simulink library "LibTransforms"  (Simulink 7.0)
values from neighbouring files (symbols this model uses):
  a0 = 0.0    (= 0)    [quake.m]    (also in rampth.m = omega^3; rspect.m = 1; displA2T.m = positT2A(zeros(ntbl, 1), dof, rh, rb, rl, canon, atype); displEnvelope.m = varargin{1}{7})
  atype = []    [displA2T.m]    (also in displEnvelope.m = varargin{1}{6}; displJacobian.m = ones(nact, 1); displT2A.m; forceA2T.m)
  canon = [linDisplCanon linVelocCanon linAccelCanon linForceCanon  		 rotDisplCanon rotVelocCanon rotAccelCanon rotForceCanon]'    [initialize.m]    (also in accelEnvelope.m = varargin{1}{4}; displEnvelope.m = varargin{1}{5}; displPivotEnvelope.m = varargin{1}{6}; forceEnvelope.m = varargin{1}{6})
  dmax = ( (stroke2 + endLength2) * lengthCanon)'    [initialize.m]
  dof = [1 2]    [initialize.m]    (also in accelEnvelope.m = varargin{1}{1}; displEnvelope.m = varargin{1}{1}; displPivotEnvelope.m = varargin{1}{1}; forceEnvelope.m = varargin{1}{2})
  ea = dcm * ea    [initialize.m]    (also in accelEnvelope.m = varargin{1}{3})
  fmax = ( area1 * areaCanon * (supplyPress-returnPress) * pressCanon)'    [initialize.m]    (also in Tutorial.m = 50; forceEnvelope.m = varargin{1}{10}; forceJacobian.m = []; forceT2A.m = [])
  gee = geeCanon / linAccelCanon * 0    (= 0)    [initialize.m]    (also in accelA2T.m; accelEnvelope.m = varargin{1}{6}; accelT2A.m)
  linAccelCanon = 9810.0    (= 9810)    [initialize.m]    (also in accelJacobian.m = canon(3); accelP2Q.m = canon(3))
  linDisplCanon = 1    [initialize.m]    (also in displJacobian.m = canon(1); velocJacobian.m = canon(1))
  linVelocCanon = 1000.0    (= 1000)    [initialize.m]    (also in forceInvJacobian.m = canon(2); velocJacobian.m = canon(2); velocP2Q.m = canon(2))
  ra = dcm * ra    [initialize.m]    (also in accelEnvelope.m = varargin{1}{2})
  rb = dcm * rb    [initialize.m]    (also in displEnvelope.m = varargin{1}{3}; displPivotEnvelope.m = varargin{1}{3}; forceEnvelope.m = varargin{1}{4}; velocEnvelope.m = varargin{1}{4})
  rh = dcm * rh    [initialize.m]    (also in displEnvelope.m = varargin{1}{2}; displPivotEnvelope.m = varargin{1}{2}; forceEnvelope.m = varargin{1}{3}; velocEnvelope.m = varargin{1}{3})
  rl = dcm * rl    [initialize.m]    (also in displEnvelope.m = varargin{1}{4}; displPivotEnvelope.m = varargin{1}{4}; forceEnvelope.m = varargin{1}{5}; velocEnvelope.m = varargin{1}{5})
  rotAccelCanon = pi/180    (= 0.0174532925199)    [initialize.m]    (also in accelJacobian.m = canon(7); accelP2Q.m = canon(7); bodyAccel.m = canon(3); eulerAccel.m = canon(3))
  rotDisplCanon = pi/180    (= 0.0174532925199)    [initialize.m]    (also in accelA2T.m = canon(5); accelP2Q.m = canon(5); accelT2A.m = canon(5); bodyAccel.m = canon(1))
  rotForceCanon = 1000    [initialize.m]    (also in forceInvJacobian.m = canon(8); forceP2Q.m = canon(8))
  rotVelocCanon = pi/180    (= 0.0174532925199)    [initialize.m]    (also in accelJacobian.m = canon(6); accelP2Q.m = canon(6); bodyAccel.m = canon(2); eulerAccel.m = canon(2))
  rows = size(header, 1)    [player.m]    (also in quake.m; savebin.m; viewer.m; accelA2T.m = size(vrot, 1))
  rpq = rpq(:)    [accelP2Q.m]    (also in displP2Q.m; forceP2Q.m; velocP2Q.m)
undefined symbols (not defined in the file or in its folder): aijac, ajac, cols, Column, D, magnitude, matrix, vector
libraries: LibTransforms x99, aerospace x9, simulink x6
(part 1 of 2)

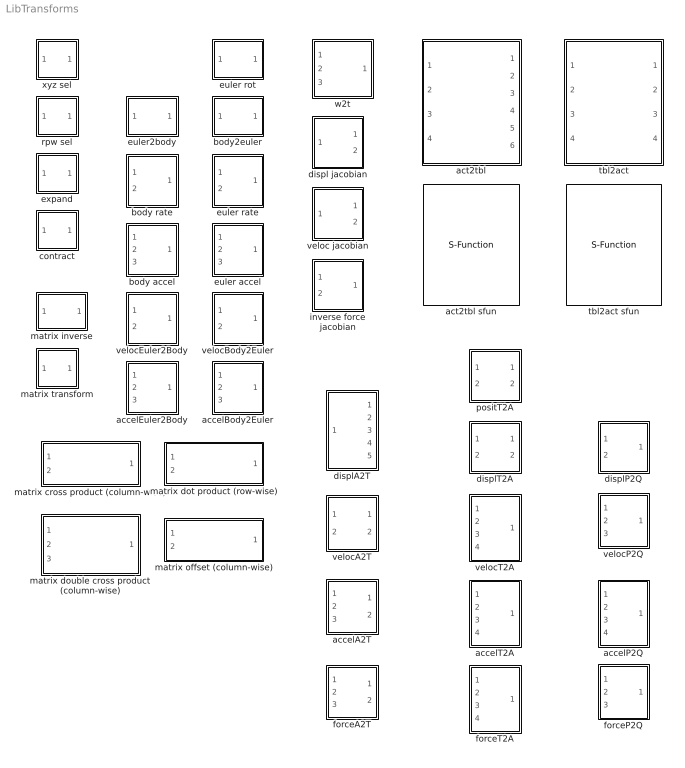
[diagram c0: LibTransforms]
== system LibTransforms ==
  accelA2T : Subsystem  mask(Accelerometer values to table acceleration tranform){dof=dof, ra=ra, ea=ea, ijac=aijac, gee=gee}
      mask prompts: dof "Degree-of-freedom indices"; ra "Accelerometer location vectors"; ea "Accelerometer orientation vectors"; ijac "Inverse acceleration jacobian"; gee "Gravity constant"
  accelBody2Euler : Subsystem  mask(Body acceleration to euler acceleration transform){dof=dof}
      mask prompts: dof "Degree-of-freedom indices"
  accelEuler2Body : Subsystem  mask(Euler acceleration to body acceleration transform){dof=dof}
      mask prompts: dof "Degree-of-freedom indices"
  accelP2Q : Subsystem  mask(Origin offset acceleration transform){dof=dof, ofst=rpq}
      mask prompts: dof "Degree-of-freedom indices"; ofst "Origin offset vector"
  accelT2A : Subsystem  mask(Table acceleration to accelerometer values tranform){dof=dof, ra=ra, ea=ea, jac=ajac, gee=gee}
      mask prompts: dof "Degree-of-freedom indices"; ra "Accelerometer location vectors"; ea "Accelerometer orientation vectors"; jac "Acceleration jacobian"; gee "Gravity constant"
  act2tbl : Subsystem  mask(Actuator to table transform){dof=dof, rh=rh, rb=rb, a0=a0, ra=ra, ea=ea, aijac=aijac, fmax=fmax, gee=gee}
      mask prompts: dof "Degree-of-freedom indices"; rh "Table pivot location vectors"; rb "Base pivot location vectors"; a0 "Actuator home position"; ra "Acceleration location vectors"; ea "Acceleration orientation vectors"; aijac "Inverse acceleration jacobian"; fmax "Actuator max forces"; gee "Gravity constant"
  act2tbl sfun : S-Function  FunctionName=Act2Tbl  Parameters=atype, nVel, nFrc, dof, rh, rb, rl, ra, ea, offset, dmax, fmax, canon, gee, action, rate, count  mask(Actuator-to-table transform){atype=atype, nVel=length(atype), nFrc=length(atype), dof=dof, rh=rh, rb=rb, rl=rl, ra=ra, ea=ea, offset=[0 0 0 0 0 0], dmax=dmax, fmax=fmax, canon=canon, gee=gee, action=1, rate=1, count=1}
      mask prompts: atype "Actuator types (1: inline; 2: pedestal-link; 3: sliding head; 4: sliding base)"; nVel "Number of velocity sensors (0 or nAct)"; nFrc "Number of force sensors (0 or nAct)"; dof "Degree-of-freedom indices (1: X; 2: Y; 3: Z; 4: Roll; 5: Pitch; 6: Yaw)"; rh "Head pivot location vectors"; rb "Base pivot location vectors"; rl "Link pivot location vectors"; ra "Accelerometer location vectors"; ea "Accelerometer orientation vectors"; offset "Coordinate system offset/rotation"; dmax "Actuator max displacements"; fmax "Actuator max forces"; canon "Canonical units"; gee "Gravity constant"; action "Jacobian update mode (0:static; 1: dyamic)"; rate "Rate type (0:body; 1:euler)"; count "Iteration count"
      mask init:
      | if nVel
      | 	velocInpName = 'velocA';
      | else
      | 	velocInpName = 'rot veloc';
      | end
  body accel : Subsystem
  body rate : Subsystem
  body2euler : Subsystem
  contract : Subsystem  mask(Linear degrees-of-freedom selector){elements=[1]}
      mask init:
      | if isempty(elements)
      | 	elements = 1;
      | end
  displ jacobian : Subsystem  mask(Displacement jacobian){dof=dof, rh=rh, rb=rb}
      mask prompts: dof "Degree-of-freedom indices"; rh "Table pivot location vectors"; rb "Base pivot location vectors"
  displA2T : Subsystem  mask(Actuator displacement to table displacement transform){dof=dof, rh=rh, rb=rb, a0=a0}
      mask prompts: dof "Degree-of-freedom indices"; rh "Table pivot location vectors"; rb "Base pivot location vectors"; a0 "Actuator home position"
  displP2Q : Subsystem  mask(Origin offset displacement transform){dof=dof, ofst=rpq}
      mask prompts: dof "Degree-of-freedom indices"; ofst "Origin offset vector"
  displT2A : Subsystem  mask(Table displacement to actuator displacement  transform){dof=dof, rh=rh, rb=rb, a0=a0}
      mask prompts: dof "Degree-of-freedom indices"; rh "Table pivot location vectors"; rb "Base pivot location vectors"; a0 "Actuator home position"
  euler accel : Subsystem
  euler rate : Subsystem
  euler rot : Subsystem
  euler2body : Subsystem
  expand : Subsystem  mask(Vector expander){size=6, elements=dof}
      mask prompts: size "Output vector size"; elements "Output vector elements (-1 for all elements)"
      mask init:
      | noElements = isempty(elements);
      | if noElements
      | 	elements = 1;
      | end
  forceA2T : Subsystem  mask(Actuator force to table force transform){dof=dof, rh=rh}
      mask prompts: dof "Degree-of-freedom indices"; rh "Table pivot location vectors"
  forceP2Q : Subsystem  mask(Origin offset force transform){dof=dof, ofst=rpq}
      mask prompts: dof "Degree-of-freedom indices"; ofst "Origin offset vector"
  forceT2A : Subsystem  mask{dof=dof, rh=rh, fmax=fmax}
      mask prompts: dof "Degree-of-freedom indices"; rh "Table pivot location vectors"; fmax "Actuator max forces"
  inverse force jacobian : Subsystem  mask(Inverse force jacobian){dof=dof, rh=rh}
      mask prompts: dof "Degree-of-freedom indices"; rh "Table pivot location vectors"
  matrix cross product (column-wise) : Subsystem  TreatAsAtomicUnit=on  mask(Matrix cross product (column-wise)){cols=size(rh,2)}
      mask prompts: cols "Number of columns"
  matrix dot product (row-wise) : Subsystem  TreatAsAtomicUnit=on  mask(Matrix dot product (row-wise)){rows=size(rh,2)}
      mask prompts: rows "Number of rows"
  matrix double cross product (column-wise) : Subsystem  TreatAsAtomicUnit=on  mask(Matrix cross product (column-wise)){cols=size(ra,2)}
      mask prompts: cols "Number of columns"
  matrix inverse : Subsystem  mask(Generalized matrix inverse){rows=rows, cols=cols, wate=[]}
      mask prompts: rows "Number of rows"; cols "Number of columns"; wate "Weight vector"
      mask init:
      | if rows < cols
      | 	c = 1;
      | 	if length(wate) == cols
      | 		w1 = diag(wate / max(wate));
      | 	else
      | 		w1 = eye(cols);
      | 	end
      | 	w2 = eye(rows);
      | elseif rows > cols
      | 	c = 2;
      | 	if length(wate) == rows
      | 		w2 = diag(wate / max(wate));
      | 	else
      | 		w2 = eye(rows);
      | 	end
      | 	w1 = eye(cols);
      | else % rows == cols
      | 	c = 3;
      | 	w1 = eye(rows);
      | 	w2 = eye(rows);
      | end
  matrix offset (column-wise) : Subsystem  TreatAsAtomicUnit=on  mask(Matrix offset (column-wise)){cols=size(rh,2)}
      mask prompts: cols "Number of columns"
  matrix transform : Subsystem  mask(Matrix transform){matrix=matrix}
      mask prompts: matrix "Transformation matrix"
  positT2A : Subsystem  mask(Table displacement to actuator position transform){dof=dof, rh=rh, rb=rb}
      mask prompts: dof "Degree-of-freedom indices"; rh "Table pivot location vectors"; rb "Base pivot location vectors"
  rpw sel : Subsystem  mask(Rotational degrees-of-freedom selector){dof=dof}
      mask prompts: dof "Degree-of-freedom indices"
      mask init:
      | elements = find(dof>3);
      | if isempty(elements)
      | 	elements = 1;
      | end
  tbl2act : Subsystem  mask(Table to actuator transform){dof=dof, rh=rh, rb=rb, a0=a0, ra=ra, ea=ea, ajac=ajac, fmax=fmax, gee=gee}
      mask prompts: dof "Degree-of-freedom indices"; rh "Table pivot location vectors"; rb "Base pivot location vectors"; a0 "Actuator home position"; ra "Accelerometer location vectors"; ea "Accelerometer orientation vectors"; ajac "Acceleration jacobian"; fmax "Actuator max forces"; gee "Gravity constant"
  tbl2act sfun : S-Function  FunctionName=Tbl2Act  Parameters=atype, nVel, nFrc, dof, rh, rb, rl, ra, ea, offset, fmax, canon, gee, action, rate  mask(Table-to-actuator transform){atype=atype, nVel=length(atype), nFrc=length(atype), dof=dof, rh=rh, rb=rb, rl=rl, ra=ra, ea=ea, offset=[0 0 0 0 0 0], fmax=fmax, canon=canon, gee=gee, action=1, rate=1}
      mask prompts: atype "Actuator types (1: inline; 2: pedestal-link; 3: sliding head; 4: sliding base)"; nVel "Number of velocity sensors (0 or nAct)"; nFrc "Number of force sensors (0 or nAct)"; dof "Degree-of-freedom indices (1: X; 2: Y; 3: Z; 4: Roll; 5: Pitch; 6: Yaw)"; rh "Head pivot location vectors"; rb "Base pivot location vectors"; rl "Link pivot location vectors"; ra "Accelerometer location vectors"; ea "Accelerometer orientation vectors"; offset "Coordinate system offset/rotation"; fmax "Actuator max forces"; canon "Canonical units"; gee "Gravity constant"; action "Jacobian update mode (0:static; 1: dyamic)"; rate "Rate type (0:body; 1:euler)"
  veloc jacobian : Subsystem  mask(Displacement jacobian){dof=dof, rh=rh, rb=rb}
      mask prompts: dof "Degree-of-freedom indices"; rh "Table pivot location vectors"; rb "Base pivot location vectors"
  velocA2T : Subsystem  mask(Table velocity to actuator velocity  transform){dof=dof, rh=rh, rb=rb}
      mask prompts: dof "Degree-of-freedom indices"; rh "Table pivot location vectors"; rb "Base pivot location vectors"
  velocBody2Euler : Subsystem  mask(Body rate to euler rate transform){dof=dof}
      mask prompts: dof "Degree-of-freedom indices"
  velocEuler2Body : Subsystem  mask(Euler rate to body rate transform){dof=dof}
      mask prompts: dof "Degree-of-freedom indices"
  velocP2Q : Subsystem  mask(Origin offset velocity transform){dof=dof, ofst=rpq}
      mask prompts: dof "Degree-of-freedom indices"; ofst "Origin offset vector"
  velocT2A : Subsystem  mask(Table velocity to actuator velocity  transform){dof=dof, rh=rh}
      mask prompts: dof "Degree-of-freedom indices"; rh "Table pivot location vectors"
  w2t : Subsystem
  xyz sel : Subsystem  mask(Linear degrees-of-freedom selector){dof=dof}
      mask prompts: dof "Degree-of-freedom indices"
      mask init:
      | elements = find(dof<=3);
      | if isempty(elements)
      | 	elements = 1;
      | end

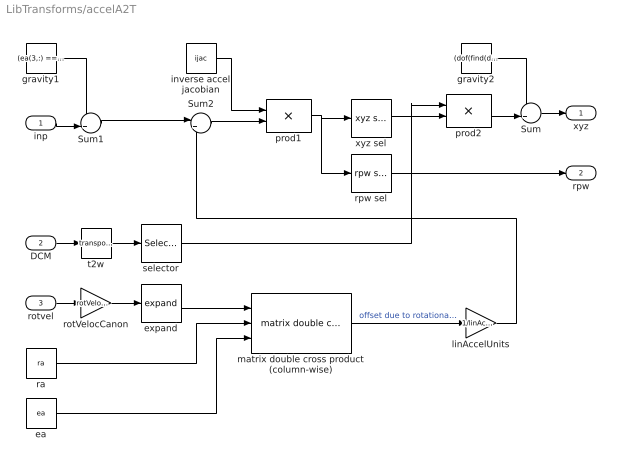
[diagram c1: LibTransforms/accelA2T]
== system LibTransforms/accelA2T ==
  inp : Inport  OutDataType=sfix(16)  OutScaling=2^0
  DCM : Inport  Port=2  OutDataType=sfix(16)  OutScaling=2^0
  rotvel : Inport  Port=3  OutDataType=sfix(16)  OutScaling=2^0
  Sum : Sum  Inputs=++|  OutDataType=sfix(16)  OutScaling=2^0
  Sum1 : Sum  Inputs=-+|  OutDataType=sfix(16)  OutScaling=2^0
  Sum2 : Sum  Inputs=|+-  OutDataType=sfix(16)  OutScaling=2^0
  ea : Constant  Value=ea  OutDataType=sfix(16)  OutScaling=2^0
  expand : LibTransforms/expand  SystemSampleTime=-1  size=3  elements=dof(find(dof>3)) - 3
  gravity1 : Constant  Value=(ea(3,:) == 1) * gee  OutDataType=sfix(16)  OutScaling=2^0
  gravity2 : Constant  Value=(dof(find(dof<=3)) == 3) * gee  OutDataType=sfix(16)  OutScaling=2^0
  inverse accel jacobian : Constant  Value=ijac  OutDataType=sfix(16)  OutScaling=2^0
  linAccelUnits : Gain  Gain=1/linAccelCanon  ParameterDataType=sfix(16)  ParameterScaling=2^0  OutDataType=sfix(16)  OutScaling=2^0
  matrix double cross product (column-wise) : LibTransforms/matrix double cross product (column-wise)  SystemSampleTime=-1  cols=size(ra,2)
  prod1 : Product  Multiplication=Matrix(*)  OutDataType=sfix(16)  OutScaling=2^0
  prod2 : Product  Multiplication=Matrix(*)  OutDataType=sfix(16)  OutScaling=2^0
  ra : Constant  Value=ra  OutDataType=sfix(16)  OutScaling=2^0
  rotVelocCanon : Gain  Gain=rotVelocCanon  ParameterDataType=sfix(16)  ParameterScaling=2^0  OutDataType=sfix(16)  OutScaling=2^0
  rpw sel : LibTransforms/rpw sel  SystemSampleTime=-1  dof=dof
  selector : Selector  NumberOfDimensions=2  InputPortWidth=3  IndexOptions=Index vector (dialog),Index vector (dialog)  Indices=dof(find(dof<=3)),dof(find(dof<=3))  OutputSizes=1
  t2w : Math  Operator=transpose  OutDataType=sfix(16)  OutScaling=2^0
  xyz sel : LibTransforms/xyz sel  SystemSampleTime=-1  dof=dof
  xyz : Outport  OutDataType=sfix(16)  OutScaling=2^0
  rpw : Outport  Port=2  OutDataType=sfix(16)  OutScaling=2^0
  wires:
  selector/1 -> prod2/1
  expand/1 -> matrix double cross product (column-wise)/1
  ea/1 -> matrix double cross product (column-wise)/3
  ra/1 -> matrix double cross product (column-wise)/2
  rotVelocCanon/1 -> expand/1
  inverse accel jacobian/1 -> prod1/1
  rotvel/1 -> rotVelocCanon/1
  gravity2/1 -> Sum/1
  gravity1/1 -> Sum1/1
  inp/1 -> Sum1/2
  Sum1/1 -> Sum2/1
  Sum2/1 -> prod1/2
  DCM/1 -> t2w/1
  xyz sel/1 -> prod2/2
  t2w/1 -> selector/1
  prod1/1 -> rpw sel/1, xyz sel/1
  prod2/1 -> Sum/2
  rpw sel/1 -> rpw/1
  Sum/1 -> xyz/1
  matrix double cross product (column-wise)/1 -> linAccelUnits/1  "offset due to rotational velocity"
  linAccelUnits/1 -> Sum2/2

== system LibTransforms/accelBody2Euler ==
  inp : Inport  OutDataType=sfix(16)  OutScaling=2^0
  rpw : Inport  Port=2  OutDataType=sfix(16)  OutScaling=2^0
  rot vel : Inport  Port=3  OutDataType=sfix(16)  OutScaling=2^0
  contract : LibTransforms/contract  SystemSampleTime=-1  elements=[dof(find(dof>3))-3]
  euler accel : LibTransforms/euler accel  SystemSampleTime=-1
  expand 1 : LibTransforms/expand  SystemSampleTime=-1  size=3  elements=dof(find(dof>3))-3
  expand 2 : LibTransforms/expand  SystemSampleTime=-1  size=3  elements=dof(find(dof>3))-3
  expand 3 : LibTransforms/expand  SystemSampleTime=-1  size=3  elements=dof(find(dof>3))-3
  out : Outport  OutDataType=sfix(16)  OutScaling=2^0
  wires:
  euler accel/1 -> contract/1
  inp/1 -> expand 1/1
  rpw/1 -> expand 2/1
  contract/1 -> out/1
  expand 1/1 -> euler accel/1
  expand 2/1 -> euler accel/2
  rot vel/1 -> expand 3/1
  expand 3/1 -> euler accel/3

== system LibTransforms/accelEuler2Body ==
  inp : Inport  OutDataType=sfix(16)  OutScaling=2^0
  rpw : Inport  Port=2  OutDataType=sfix(16)  OutScaling=2^0
  rot vel : Inport  Port=3  OutDataType=sfix(16)  OutScaling=2^0
  body accel : LibTransforms/body accel  SystemSampleTime=-1
  contract : LibTransforms/contract  SystemSampleTime=-1  elements=[dof(find(dof>3))-3]
  expand 1 : LibTransforms/expand  SystemSampleTime=-1  size=3  elements=dof(find(dof>3))-3
  expand 2 : LibTransforms/expand  SystemSampleTime=-1  size=3  elements=dof(find(dof>3))-3
  expand 3 : LibTransforms/expand  SystemSampleTime=-1  size=3  elements=dof(find(dof>3))-3
  out : Outport  OutDataType=sfix(16)  OutScaling=2^0
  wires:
  expand 3/1 -> body accel/3
  rot vel/1 -> expand 3/1
  expand 2/1 -> body accel/2
  expand 1/1 -> body accel/1
  contract/1 -> out/1
  rpw/1 -> expand 2/1
  inp/1 -> expand 1/1
  body accel/1 -> contract/1

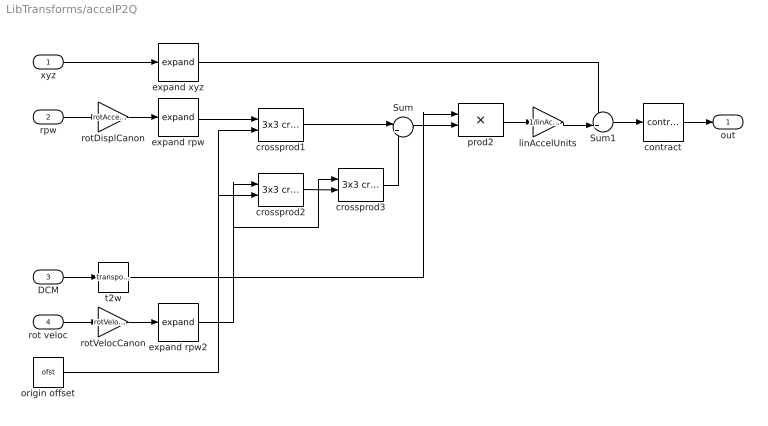
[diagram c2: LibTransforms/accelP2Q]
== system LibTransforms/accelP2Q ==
  xyz : Inport  OutDataType=sfix(16)  OutScaling=2^0
  rpw : Inport  Port=2  OutDataType=sfix(16)  OutScaling=2^0
  DCM : Inport  Port=3  OutDataType=sfix(16)  OutScaling=2^0
  rot veloc : Inport  Port=4  OutDataType=sfix(16)  OutScaling=2^0
  Sum : Sum  Inputs=|++  OutDataType=sfix(16)  OutScaling=2^0
  Sum1 : Sum  Inputs=++|  OutDataType=sfix(16)  OutScaling=2^0
  contract : LibTransforms/contract  SystemSampleTime=-1  elements=dof(find(dof<=3))
  crossprod1 : aerospace/Axes Transformations/3x3 cross product  SystemSampleTime=-1
  crossprod2 : aerospace/Axes Transformations/3x3 cross product  SystemSampleTime=-1
  crossprod3 : aerospace/Axes Transformations/3x3 cross product  SystemSampleTime=-1
  expand rpw : LibTransforms/expand  SystemSampleTime=-1  size=3  elements=dof(find(dof>3)) - 3
  expand rpw2 : LibTransforms/expand  SystemSampleTime=-1  size=3  elements=dof(find(dof>3)) - 3
  expand xyz : LibTransforms/expand  SystemSampleTime=-1  size=3  elements=dof(find(dof<=3))
  linAccelUnits : Gain  Gain=1/linAccelCanon  ParameterDataType=sfix(16)  ParameterScaling=2^0  OutDataType=sfix(16)  OutScaling=2^0
  origin offset : Constant  Value=ofst  OutDataType=sfix(16)  OutScaling=2^0
  prod2 : Product  Multiplication=Matrix(*)  OutDataType=sfix(16)  OutScaling=2^0
  rotDisplCanon : Gain  Gain=rotAccelCanon  ParameterDataType=sfix(16)  ParameterScaling=2^0  OutDataType=sfix(16)  OutScaling=2^0
  rotVelocCanon : Gain  Gain=rotVelocCanon  ParameterDataType=sfix(16)  ParameterScaling=2^0  OutDataType=sfix(16)  OutScaling=2^0
  t2w : Math  Operator=transpose  OutDataType=sfix(16)  OutScaling=2^0
  out : Outport  OutDataType=sfix(16)  OutScaling=2^0
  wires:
  crossprod1/1 -> Sum/1
  crossprod3/1 -> Sum/2
  Sum1/1 -> contract/1
  crossprod2/1 -> crossprod3/2
  Sum/1 -> prod2/2
  origin offset/1 -> crossprod1/2, crossprod2/2
  rotDisplCanon/1 -> expand rpw/1
  rpw/1 -> rotDisplCanon/1
  t2w/1 -> prod2/1
  xyz/1 -> expand xyz/1
  rot veloc/1 -> rotVelocCanon/1
  DCM/1 -> t2w/1
  rotVelocCanon/1 -> expand rpw2/1
  linAccelUnits/1 -> Sum1/2
  expand rpw2/1 -> crossprod3/1, crossprod2/1
  expand rpw/1 -> crossprod1/1
  expand xyz/1 -> Sum1/1
  prod2/1 -> linAccelUnits/1
  contract/1 -> out/1

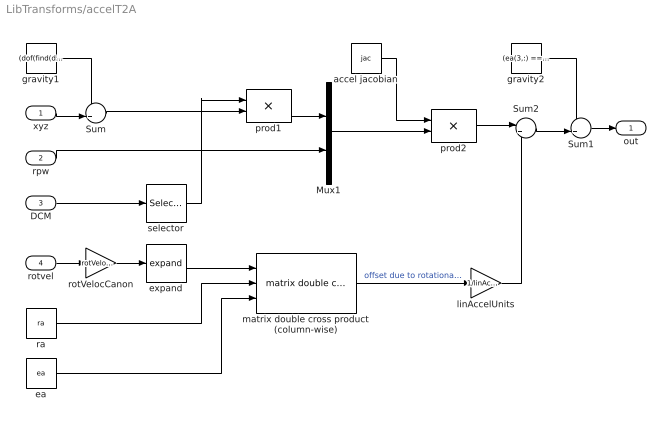
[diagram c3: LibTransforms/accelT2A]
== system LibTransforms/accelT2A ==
  xyz : Inport  OutDataType=sfix(16)  OutScaling=2^0
  rpw : Inport  Port=2  OutDataType=sfix(16)  OutScaling=2^0
  DCM : Inport  Port=3  OutDataType=sfix(16)  OutScaling=2^0
  rotvel : Inport  Port=4  OutDataType=sfix(16)  OutScaling=2^0
  Mux1 : Mux  Inputs=2
  Sum : Sum  Inputs=-+|  OutDataType=sfix(16)  OutScaling=2^0
  Sum1 : Sum  Inputs=++|  OutDataType=sfix(16)  OutScaling=2^0
  Sum2 : Sum  Inputs=|++  OutDataType=sfix(16)  OutScaling=2^0
  accel jacobian : Constant  Value=jac  OutDataType=sfix(16)  OutScaling=2^0
  ea : Constant  Value=ea  OutDataType=sfix(16)  OutScaling=2^0
  expand : LibTransforms/expand  SystemSampleTime=-1  size=3  elements=dof(find(dof>3)) - 3
  gravity1 : Constant  Value=(dof(find(dof<=3)) == 3) * gee  OutDataType=sfix(16)  OutScaling=2^0
  gravity2 : Constant  Value=(ea(3,:) == 1) * gee  OutDataType=sfix(16)  OutScaling=2^0
  linAccelUnits : Gain  Gain=1/linAccelCanon  ParameterDataType=sfix(16)  ParameterScaling=2^0  OutDataType=sfix(16)  OutScaling=2^0
  matrix double cross product (column-wise) : LibTransforms/matrix double cross product (column-wise)  SystemSampleTime=-1  cols=size(ra,2)
  prod1 : Product  Multiplication=Matrix(*)  OutDataType=sfix(16)  OutScaling=2^0
  prod2 : Product  Multiplication=Matrix(*)  OutDataType=sfix(16)  OutScaling=2^0
  ra : Constant  Value=ra  OutDataType=sfix(16)  OutScaling=2^0
  rotVelocCanon : Gain  Gain=rotVelocCanon  ParameterDataType=sfix(16)  ParameterScaling=2^0  OutDataType=sfix(16)  OutScaling=2^0
  selector : Selector  NumberOfDimensions=2  InputPortWidth=3  IndexOptions=Index vector (dialog),Index vector (dialog)  Indices=dof(find(dof<=3)),dof(find(dof<=3))  OutputSizes=1
  out : Outport  OutDataType=sfix(16)  OutScaling=2^0
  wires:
  selector/1 -> prod1/1
  expand/1 -> matrix double cross product (column-wise)/1
  rotVelocCanon/1 -> expand/1
  ea/1 -> matrix double cross product (column-wise)/3
  ra/1 -> matrix double cross product (column-wise)/2
  gravity2/1 -> Sum1/1
  Sum1/1 -> out/1
  gravity1/1 -> Sum/1
  xyz/1 -> Sum/2
  Sum/1 -> prod1/2
  DCM/1 -> selector/1
  rotvel/1 -> rotVelocCanon/1
  rpw/1 -> Mux1/2
  Sum2/1 -> Sum1/2
  matrix double cross product (column-wise)/1 -> linAccelUnits/1  "offset due to rotational velocity"
  prod1/1 -> Mux1/1
  accel jacobian/1 -> prod2/1
  Mux1/1 -> prod2/2
  prod2/1 -> Sum2/1
  linAccelUnits/1 -> Sum2/2

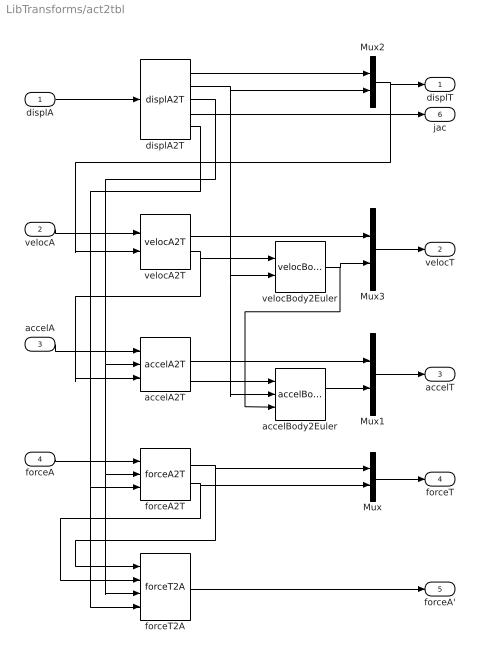
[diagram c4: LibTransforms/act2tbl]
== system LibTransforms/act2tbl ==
  displA : Inport  OutDataType=sfix(16)  OutScaling=2^0
  velocA : Inport  Port=2  OutDataType=sfix(16)  OutScaling=2^0
  accelA : Inport  Port=3  OutDataType=sfix(16)  OutScaling=2^0
  forceA : Inport  Port=4  OutDataType=sfix(16)  OutScaling=2^0
  Mux{,1..3} (4 alike) : Mux  Inputs=2
  accelA2T : LibTransforms/accelA2T  SystemSampleTime=-1  dof=dof  ra=ra  ea=ea  ijac=aijac  gee=gee
  accelBody2Euler : LibTransforms/accelBody2Euler  SystemSampleTime=-1  dof=dof
  displA2T : LibTransforms/displA2T  SystemSampleTime=-1  dof=dof  rh=rh  rb=rb  a0=a0
  forceA2T : LibTransforms/forceA2T  SystemSampleTime=-1  dof=dof  rh=rh
  forceT2A : LibTransforms/forceT2A  SystemSampleTime=-1  dof=dof  rh=rh  fmax=fmax
  velocA2T : LibTransforms/velocA2T  SystemSampleTime=-1  dof=dof  rh=rh  rb=rb
  velocBody2Euler : LibTransforms/velocBody2Euler  SystemSampleTime=-1  dof=dof
  displT : Outport  OutDataType=sfix(16)  OutScaling=2^0
  velocT : Outport  Port=2  OutDataType=sfix(16)  OutScaling=2^0
  accelT : Outport  Port=3  OutDataType=sfix(16)  OutScaling=2^0
  forceT : Outport  Port=4  OutDataType=sfix(16)  OutScaling=2^0
  forceA' : Outport  Port=5  OutDataType=sfix(16)  OutScaling=2^0
  jac : Outport  Port=6  OutDataType=sfix(16)  OutScaling=2^0
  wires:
  velocBody2Euler/1 -> Mux3/2, accelBody2Euler/3
  displA2T/3 -> accelA2T/2, forceA2T/2, forceT2A/3
  accelA/1 -> accelA2T/1
  displA2T/1 -> Mux2/1
  displA2T/2 -> accelBody2Euler/2, velocBody2Euler/2, Mux2/2
  Mux2/1 -> velocA2T/2, displT/1
  accelA2T/1 -> Mux1/1
  displA/1 -> displA2T/1
  forceA2T/1 -> Mux/1, forceT2A/1
  forceA2T/2 -> Mux/2, forceT2A/2
  forceA/1 -> forceA2T/1
  Mux1/1 -> accelT/1
  Mux/1 -> forceT/1
  displA2T/4 -> jac/1
  displA2T/5 -> forceA2T/3, forceT2A/4
  accelA2T/2 -> accelBody2Euler/1
  accelBody2Euler/1 -> Mux1/2
  forceT2A/1 -> forceA'/1
  Mux3/1 -> velocT/1
  velocA2T/1 -> Mux3/1
  velocA2T/2 -> accelA2T/3, velocBody2Euler/1
  velocA/1 -> velocA2T/1

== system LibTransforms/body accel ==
  inp : Inport  OutDataType=sfix(16)  OutScaling=2^0
  rpw : Inport  Port=2  OutDataType=sfix(16)  OutScaling=2^0
  rot vel : Inport  Port=3  OutDataType=sfix(16)  OutScaling=2^0
  Mux2 : Mux  Inputs=2
  Sum2 : Sum  Inputs=|++  OutDataType=sfix(16)  OutScaling=2^0
  euler2body : LibTransforms/euler2body  SystemSampleTime=-1
  prod : Product  Multiplication=Matrix(*)  OutDataType=sfix(16)  OutScaling=2^0
  rate cross terms : Subsystem
  rotAccelUnits : Gain  Gain=1/rotAccelCanon  ParameterDataType=sfix(16)  ParameterScaling=2^0  OutDataType=sfix(16)  OutScaling=2^0
  rotDisplCanon : Gain  Gain=rotDisplCanon  ParameterDataType=sfix(16)  ParameterScaling=2^0  OutDataType=sfix(16)  OutScaling=2^0
  rotVelocCanon : Gain  Gain=rotVelocCanon  ParameterDataType=sfix(16)  ParameterScaling=2^0  OutDataType=sfix(16)  OutScaling=2^0
  out : Outport  OutDataType=sfix(16)  OutScaling=2^0
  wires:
  Mux2/1 -> rate cross terms/1(inp)
  rate cross terms/1(out) -> rotAccelUnits/1
  Sum2/1 -> out/1  "body accels"
  prod/1 -> Sum2/1
  rot vel/1 -> rotVelocCanon/1  "euler rates"
  euler2body/1 -> prod/1
  rpw/1 -> rotDisplCanon/1  "euler angles"
  inp/1 -> prod/2  "euler accels"
  rotDisplCanon/1 -> euler2body/1, Mux2/1
  rotVelocCanon/1 -> Mux2/2
  rotAccelUnits/1 -> Sum2/2

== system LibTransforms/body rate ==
  inp : Inport  OutDataType=sfix(16)  OutScaling=2^0
  rpw : Inport  Port=2  OutDataType=sfix(16)  OutScaling=2^0
  euler2body : LibTransforms/euler2body  SystemSampleTime=-1
  prod : Product  Multiplication=Matrix(*)  OutDataType=sfix(16)  OutScaling=2^0
  rotDisplCanon : Gain  Gain=rotDisplCanon  ParameterDataType=sfix(16)  ParameterScaling=2^0  OutDataType=sfix(16)  OutScaling=2^0
  out : Outport  OutDataType=sfix(16)  OutScaling=2^0
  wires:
  rotDisplCanon/1 -> euler2body/1
  inp/1 -> prod/2  "euler rates"
  prod/1 -> out/1  "body rates"
  rpw/1 -> rotDisplCanon/1  "euler angles"
  euler2body/1 -> prod/1

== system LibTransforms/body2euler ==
  rpw : Inport  OutDataType=sfix(16)  OutScaling=2^0
  11 : Fcn  Expr=1
  12 : Fcn  Expr=sin(u[1])*tan(u[2])
  13 : Fcn  Expr=cos(u[1])*tan(u[2])
  21 : Fcn  Expr=0
  22 : Fcn  Expr=cos(u[1])
  23 : Fcn  Expr=-sin(u[1])
  31 : Fcn  Expr=0
  32 : Fcn  Expr=sin(u[1])/cos(u[2])
  33 : Fcn  Expr=cos(u[1])/cos(u[2])
  9x1->3x3 : Reshape  OutputDimensionality=Customize  OutputDimensions=[3,3]
  Mux2 : Mux  Orientation=down  Inputs=9
  out : Outport  OutDataType=sfix(16)  OutScaling=2^0
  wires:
  9x1->3x3/1 -> out/1
  11/1 -> Mux2/1
  21/1 -> Mux2/2
  31/1 -> Mux2/3
  rpw/1 -> 31/1, 21/1, 11/1, 32/1, 22/1, 12/1, 33/1, 23/1, 13/1
  12/1 -> Mux2/4
  22/1 -> Mux2/5
  32/1 -> Mux2/6
  Mux2/1 -> 9x1->3x3/1
  13/1 -> Mux2/7
  23/1 -> Mux2/8
  33/1 -> Mux2/9

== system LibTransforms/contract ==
  inp : Inport  OutDataType=sfix(16)  OutScaling=2^0
  Selector : Selector  IndexOptions=Index vector (dialog)  Indices=elements  OutputSizes=1
  out : Outport  OutDataType=sfix(16)  OutScaling=2^0
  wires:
  inp/1 -> Selector/1
  Selector/1 -> out/1

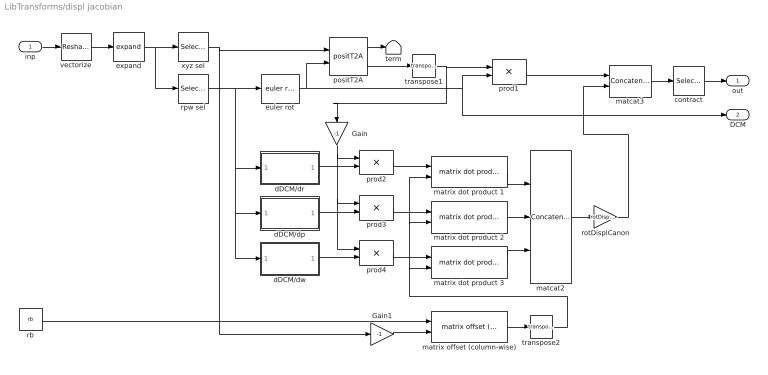
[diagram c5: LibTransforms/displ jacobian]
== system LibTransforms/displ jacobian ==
  inp : Inport  OutDataType=sfix(16)  OutScaling=2^0
  Gain : Gain  Orientation=down  Gain=-1  ParameterDataType=sfix(16)  ParameterScaling=2^0  OutDataType=sfix(16)  OutScaling=2^0
  Gain1 : Gain  Gain=-1  ParameterDataType=sfix(16)  ParameterScaling=2^0  OutDataType=sfix(16)  OutScaling=2^0
  contract : Selector  NumberOfDimensions=2  InputPortWidth=3  IndexOptions=Select all,Index vector (dialog)  Indices=-1,dof  OutputSizes=1
  dDCM/dp : Subsystem
  dDCM/dr : Subsystem
  dDCM/dw : Subsystem
  euler rot : LibTransforms/euler rot  SystemSampleTime=-1
  expand : LibTransforms/expand  SystemSampleTime=-1  size=6  elements=dof
  matcat2 : Concatenate  NumInputs=3  Mode=Multidimensional array  ConcatenateDimension=2
  matcat3 : Concatenate  Mode=Multidimensional array  ConcatenateDimension=2
  matrix dot product 1 : LibTransforms/matrix dot product (row-wise)  SystemSampleTime=-1  rows=size(rh,2)
  matrix dot product 2 : LibTransforms/matrix dot product (row-wise)  SystemSampleTime=-1  rows=size(rh,2)
  matrix dot product 3 : LibTransforms/matrix dot product (row-wise)  SystemSampleTime=-1  rows=size(rh,2)
  matrix offset (column-wise) : LibTransforms/matrix offset (column-wise)  SystemSampleTime=-1  cols=size(rh,2)
  positT2A : LibTransforms/positT2A  SystemSampleTime=-1  dof=1:6  rh=rh  rb=rb
  prod{1..4} (4 alike) : Product  Multiplication=Matrix(*)  OutDataType=sfix(16)  OutScaling=2^0
  rb : Constant  Value=rb  OutDataType=sfix(16)  OutScaling=2^0
  rotDisplCanon : Gain  Gain=rotDisplCanon  ParameterDataType=sfix(16)  ParameterScaling=2^0  OutDataType=sfix(16)  OutScaling=2^0
  rpw sel : Selector  IndexOptions=Index vector (dialog)  Indices=[4 5 6]  OutputSizes=1
  term : Terminator
  transpose1 : Math  Operator=transpose  OutDataType=sfix(16)  OutScaling=2^0
  transpose2 : Math  Operator=transpose  OutDataType=sfix(16)  OutScaling=2^0
  vectorize : Reshape  OutputDimensionality=Column vector (2-D)  OutputDimensions=[3,3]
  xyz sel : Selector  IndexOptions=Index vector (dialog)  Indices=[1 2 3]  OutputSizes=1
  out : Outport  OutDataType=sfix(16)  OutScaling=2^0
  DCM : Outport  Port=2  OutDataType=sfix(16)  OutScaling=2^0
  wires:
  vectorize/1 -> expand/1
  contract/1 -> out/1
  expand/1 -> xyz sel/1, rpw sel/1
  transpose1/1 -> Gain/1, prod1/1
  positT2A/2 -> transpose1/1
  Gain/1 -> prod2/1, prod3/1, prod4/1
  matcat3/1 -> contract/1
  prod1/1 -> matcat3/1
  matcat2/1 -> rotDisplCanon/1
  prod4/1 -> matrix dot product 3/1
  prod3/1 -> matrix dot product 2/1
  prod2/1 -> matrix dot product 1/1
  matrix offset (column-wise)/1 -> transpose2/1
  dDCM/dp/1(dDCM/dp) -> prod3/2
  dDCM/dw/1(dDCM/dw) -> prod4/2
  dDCM/dr/1(dDCM/dr) -> prod2/2
  positT2A/1 -> term/1
  xyz sel/1 -> Gain1/1, positT2A/1
  euler rot/1 -> DCM/1, prod1/2, positT2A/2
  rpw sel/1 -> dDCM/dr/1(rpw), dDCM/dp/1(rpw), dDCM/dw/1(rpw), euler rot/1
  inp/1 -> vectorize/1
  matrix dot product 1/1 -> matcat2/1
  matrix dot product 2/1 -> matcat2/2
  matrix dot product 3/1 -> matcat2/3
  rotDisplCanon/1 -> matcat3/2
  transpose2/1 -> matrix dot product 1/2, matrix dot product 2/2, matrix dot product 3/2
  Gain1/1 -> matrix offset (column-wise)/2
  rb/1 -> matrix offset (column-wise)/1

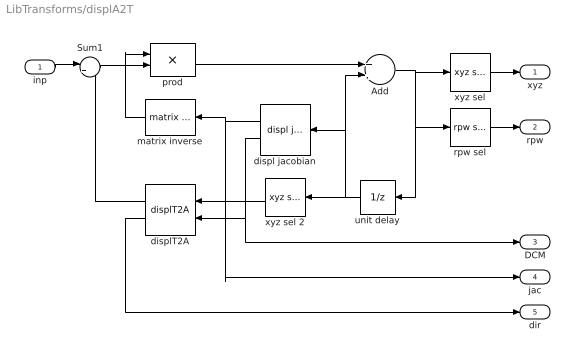
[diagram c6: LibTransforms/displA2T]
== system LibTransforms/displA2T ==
  inp : Inport  OutDataType=sfix(16)  OutScaling=2^0
  Add : Sum  OutDataType=sfix(16)  OutScaling=2^-10
  Sum1 : Sum  Inputs=|+-  OutDataType=sfix(16)  OutScaling=2^0
  displ jacobian : LibTransforms/displ jacobian  Orientation=left  SystemSampleTime=-1  dof=dof  rh=rh  rb=rb
  displT2A : LibTransforms/displT2A  Orientation=left  SystemSampleTime=-1  dof=dof  rh=rh  rb=rb  a0=a0
  matrix inverse : LibTransforms/matrix inverse  Orientation=left  SystemSampleTime=-1  rows=size(rh, 2)  cols=length(dof)  wate=[]
  prod : Product  Multiplication=Matrix(*)  OutDataType=sfix(16)  OutScaling=2^0
  rpw sel : LibTransforms/rpw sel  SystemSampleTime=-1  dof=dof
  unit delay : UnitDelay  Orientation=left  SampleTime=-1
  xyz sel : LibTransforms/xyz sel  SystemSampleTime=-1  dof=dof
  xyz sel 2 : LibTransforms/xyz sel  Orientation=left  SystemSampleTime=-1  dof=dof
  xyz : Outport  OutDataType=sfix(16)  OutScaling=2^0
  rpw : Outport  Port=2  OutDataType=sfix(16)  OutScaling=2^0
  DCM : Outport  Port=3  OutDataType=sfix(16)  OutScaling=2^0
  jac : Outport  Port=4  OutDataType=sfix(16)  OutScaling=2^0
  dir : Outport  Port=5  OutDataType=sfix(16)  OutScaling=2^0
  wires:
  displT2A/2 -> dir/1
  displT2A/1 -> Sum1/2
  Sum1/1 -> prod/2
  unit delay/1 -> xyz sel 2/1, displ jacobian/1, Add/2
  inp/1 -> Sum1/1
  Add/1 -> xyz sel/1, rpw sel/1, unit delay/1
  matrix inverse/1 -> prod/1
  displ jacobian/2 -> displT2A/2, DCM/1
  displ jacobian/1 -> matrix inverse/1, jac/1
  xyz sel 2/1 -> displT2A/1
  prod/1 -> Add/1
  xyz sel/1 -> xyz/1
  rpw sel/1 -> rpw/1

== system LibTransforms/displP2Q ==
  xyz : Inport  OutDataType=sfix(16)  OutScaling=2^0
  DCM : Inport  Port=2  OutDataType=sfix(16)  OutScaling=2^0
  Sum1 : Sum  Inputs=++-  OutDataType=sfix(16)  OutScaling=2^0
  contract : LibTransforms/contract  SystemSampleTime=-1  elements=dof(find(dof<=3))
  expand : LibTransforms/expand  SystemSampleTime=-1  size=3  elements=dof(find(dof<=3))
  origin offset : Constant  Value=ofst  OutDataType=sfix(16)  OutScaling=2^0
  prod : Product  Multiplication=Matrix(*)  OutDataType=sfix(16)  OutScaling=2^0
  t2w : Math  Operator=transpose  OutDataType=sfix(16)  OutScaling=2^0
  out : Outport  OutDataType=sfix(16)  OutScaling=2^0
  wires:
  t2w/1 -> prod/1
  DCM/1 -> t2w/1
  origin offset/1 -> prod/2, Sum1/3
  xyz/1 -> expand/1
  prod/1 -> Sum1/2
  Sum1/1 -> contract/1
  expand/1 -> Sum1/1
  contract/1 -> out/1

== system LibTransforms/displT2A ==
  xyz : Inport  OutDataType=sfix(16)  OutScaling=2^0
  DCM : Inport  Port=2  OutDataType=sfix(16)  OutScaling=2^0
  Sum6 : Sum  Inputs=|+-  OutDataType=sfix(16)  OutScaling=2^0
  a0 : Constant  Value=a0  OutDataType=sfix(16)  OutScaling=2^0
  positT2A : LibTransforms/positT2A  SystemSampleTime=-1  dof=dof  rh=rh  rb=rb
  out : Outport  OutDataType=sfix(16)  OutScaling=2^0
  dir : Outport  Port=2  OutDataType=sfix(16)  OutScaling=2^0
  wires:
  Sum6/1 -> out/1
  a0/1 -> Sum6/2
  xyz/1 -> positT2A/1
  DCM/1 -> positT2A/2
  positT2A/2 -> dir/1
  positT2A/1 -> Sum6/1

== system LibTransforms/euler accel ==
  inp : Inport  OutDataType=sfix(16)  OutScaling=2^0
  rpw : Inport  Port=2  OutDataType=sfix(16)  OutScaling=2^0
  rot vel : Inport  Port=3  OutDataType=sfix(16)  OutScaling=2^0
  Mux2 : Mux  Inputs=2
  Sum2 : Sum  Inputs=|++  OutDataType=sfix(16)  OutScaling=2^0
  body2euler : LibTransforms/body2euler  SystemSampleTime=-1
  prod : Product  Multiplication=Matrix(*)  OutDataType=sfix(16)  OutScaling=2^0
  rate cross terms : Subsystem
  rotAccelUnits : Gain  Gain=1/rotAccelCanon  ParameterDataType=sfix(16)  ParameterScaling=2^0  OutDataType=sfix(16)  OutScaling=2^0
  rotDisplCanon : Gain  Gain=rotDisplCanon  ParameterDataType=sfix(16)  ParameterScaling=2^0  OutDataType=sfix(16)  OutScaling=2^0
  rotVelocCanon : Gain  Gain=rotVelocCanon  ParameterDataType=sfix(16)  ParameterScaling=2^0  OutDataType=sfix(16)  OutScaling=2^0
  out : Outport  OutDataType=sfix(16)  OutScaling=2^0
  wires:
  rotDisplCanon/1 -> body2euler/1, Mux2/1
  inp/1 -> prod/2  "body accels"
  rpw/1 -> rotDisplCanon/1  "euler angles"
  body2euler/1 -> prod/1
  rot vel/1 -> rotVelocCanon/1  "euler rates"
  prod/1 -> Sum2/1
  Sum2/1 -> out/1  "euler accels"
  rate cross terms/1(out) -> rotAccelUnits/1
  Mux2/1 -> rate cross terms/1(inp)
  rotVelocCanon/1 -> Mux2/2
  rotAccelUnits/1 -> Sum2/2

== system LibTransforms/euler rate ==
  inp : Inport  OutDataType=sfix(16)  OutScaling=2^0
  rpw : Inport  Port=2  OutDataType=sfix(16)  OutScaling=2^0
  body2euler : LibTransforms/body2euler  SystemSampleTime=-1
  prod : Product  Multiplication=Matrix(*)  OutDataType=sfix(16)  OutScaling=2^0
  rotDisplCanon : Gain  Gain=rotDisplCanon  ParameterDataType=sfix(16)  ParameterScaling=2^0  OutDataType=sfix(16)  OutScaling=2^0
  out : Outport  OutDataType=sfix(16)  OutScaling=2^0
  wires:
  rotDisplCanon/1 -> body2euler/1
  inp/1 -> prod/2  "body rates"
  prod/1 -> out/1  "euler rates"
  rpw/1 -> rotDisplCanon/1  "euler angles"
  body2euler/1 -> prod/1

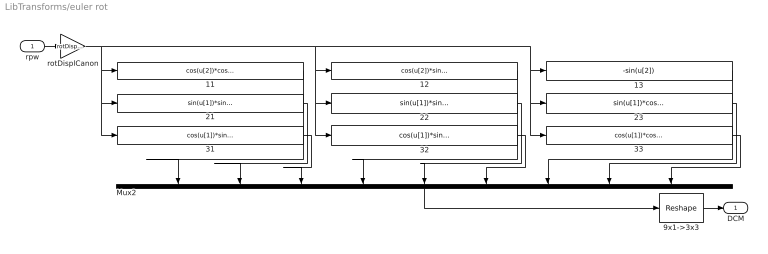
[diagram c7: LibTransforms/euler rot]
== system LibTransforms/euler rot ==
  rpw : Inport  OutDataType=sfix(16)  OutScaling=2^0
  11 : Fcn  Expr=cos(u[2])*cos(u[3])
  12 : Fcn  Expr=cos(u[2])*sin(u[3])
  13 : Fcn  Expr=-sin(u[2])
  21 : Fcn  Expr=sin(u[1])*sin(u[2])*cos(u[3])-cos(u[1])*sin(u[3])
  22 : Fcn  Expr=sin(u[1])*sin(u[2])*sin(u[3])+cos(u[1])*cos(u[3])
  23 : Fcn  Expr=sin(u[1])*cos(u[2])
  31 : Fcn  Expr=cos(u[1])*sin(u[2])*cos(u[3])+sin(u[1])*sin(u[3])
  32 : Fcn  Expr=cos(u[1])*sin(u[2])*sin(u[3])-sin(u[1])*cos(u[3])
  33 : Fcn  Expr=cos(u[1])*cos(u[2])
  9x1->3x3 : Reshape  OutputDimensionality=Customize  OutputDimensions=[3,3]
  Mux2 : Mux  Orientation=down  Inputs=9
  rotDisplCanon : Gain  Gain=rotDisplCanon  ParameterDataType=sfix(16)  ParameterScaling=2^0  OutDataType=sfix(16)  OutScaling=2^0
  DCM : Outport  OutDataType=sfix(16)  OutScaling=2^0
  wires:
  rotDisplCanon/1 -> 31/1, 21/1, 11/1, 32/1, 22/1, 12/1, 33/1, 23/1, 13/1
  9x1->3x3/1 -> DCM/1
  11/1 -> Mux2/1
  21/1 -> Mux2/2
  31/1 -> Mux2/3
  rpw/1 -> rotDisplCanon/1
  12/1 -> Mux2/4
  22/1 -> Mux2/5
  32/1 -> Mux2/6
  Mux2/1 -> 9x1->3x3/1
  13/1 -> Mux2/7
  23/1 -> Mux2/8
  33/1 -> Mux2/9

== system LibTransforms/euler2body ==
  rpw : Inport  OutDataType=sfix(16)  OutScaling=2^0
  11 : Fcn  Expr=1
  12 : Fcn  Expr=0
  13 : Fcn  Expr=-sin(u[2])
  21 : Fcn  Expr=0
  22 : Fcn  Expr=cos(u[1])
  23 : Fcn  Expr=sin(u[1])*cos(u[2])
  31 : Fcn  Expr=0
  32 : Fcn  Expr=-sin(u[1])
  33 : Fcn  Expr=cos(u[1])*cos(u[2])
  9x1->3x3 : Reshape  OutputDimensionality=Customize  OutputDimensions=[3,3]
  Mux2 : Mux  Orientation=down  Inputs=9
  out : Outport  OutDataType=sfix(16)  OutScaling=2^0
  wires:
  9x1->3x3/1 -> out/1
  11/1 -> Mux2/1
  21/1 -> Mux2/2
  31/1 -> Mux2/3
  rpw/1 -> 31/1, 21/1, 11/1, 32/1, 22/1, 12/1, 33/1, 23/1, 13/1
  12/1 -> Mux2/4
  22/1 -> Mux2/5
  32/1 -> Mux2/6
  Mux2/1 -> 9x1->3x3/1
  13/1 -> Mux2/7
  23/1 -> Mux2/8
  33/1 -> Mux2/9

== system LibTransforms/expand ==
  inp : Inport  OutDataType=sfix(16)  OutScaling=2^0
  Assignment : Assignment  IndexOptions=Index vector (dialog)  Indices=elements  OutputSizes=[1 1]
  bypass : MultiPortSwitch  Inputs=2  zeroidx=on  OutDataType=sfix(16)  OutScaling=2^0
  noElements : Constant  Value=noElements  OutDataType=sfix(16)  OutScaling=2^0
  zeros : Constant  Value=zeros(size,1)  OutDataType=sfix(16)  OutScaling=2^0
  out : Outport  OutDataType=sfix(16)  OutScaling=2^0
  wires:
  Assignment/1 -> bypass/2
  noElements/1 -> bypass/1
  bypass/1 -> out/1
  inp/1 -> Assignment/2
  zeros/1 -> bypass/3, Assignment/1

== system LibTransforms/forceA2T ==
  inp : Inport  OutDataType=sfix(16)  OutScaling=2^0
  DCM : Inport  Port=2  OutDataType=sfix(16)  OutScaling=2^0
  dir : Inport  Port=3  OutDataType=sfix(16)  OutScaling=2^0
  inverse force jacobian : LibTransforms/inverse force jacobian  SystemSampleTime=-1  dof=dof  rh=rh
  prod2 : Product  Multiplication=Matrix(*)  OutDataType=sfix(16)  OutScaling=2^0
  rpw sel : LibTransforms/rpw sel  SystemSampleTime=-1  dof=dof
  xyz sel : LibTransforms/xyz sel  SystemSampleTime=-1  dof=dof
  xyz : Outport  OutDataType=sfix(16)  OutScaling=2^0
  rpw : Outport  Port=2  OutDataType=sfix(16)  OutScaling=2^0
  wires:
  dir/1 -> inverse force jacobian/1  "ebt_t"
  inverse force jacobian/1 -> prod2/1
  DCM/1 -> inverse force jacobian/2
  xyz sel/1 -> xyz/1
  rpw sel/1 -> rpw/1
  inp/1 -> prod2/2
  prod2/1 -> rpw sel/1, xyz sel/1

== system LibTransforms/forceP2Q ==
  xyz : Inport  OutDataType=sfix(16)  OutScaling=2^0
  rpw : Inport  Port=2  OutDataType=sfix(16)  OutScaling=2^0
  DCM : Inport  Port=3  OutDataType=sfix(16)  OutScaling=2^0
  Sum : Sum  Inputs=++|  OutDataType=sfix(16)  OutScaling=2^0
  contract : LibTransforms/contract  SystemSampleTime=-1  elements=dof(find(dof>3))-3
  crossprod : aerospace/Axes Transformations/3x3 cross product  SystemSampleTime=-1
  expand rpw : LibTransforms/expand  SystemSampleTime=-1  size=3  elements=dof(find(dof>3)) - 3
  expand xyz : LibTransforms/expand  SystemSampleTime=-1  size=3  elements=dof(find(dof<=3))
  origin offset : Constant  Value=ofst  OutDataType=sfix(16)  OutScaling=2^0
  prod : Product  Multiplication=Matrix(*)  OutDataType=sfix(16)  OutScaling=2^0
  rotForceUnits : Gain  Gain=1/rotForceCanon  ParameterDataType=sfix(16)  ParameterScaling=2^0  OutDataType=sfix(16)  OutScaling=2^0
  out : Outport  OutDataType=sfix(16)  OutScaling=2^0
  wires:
  origin offset/1 -> crossprod/2
  prod/1 -> crossprod/1
  DCM/1 -> prod/1
  xyz/1 -> expand xyz/1
  rotForceUnits/1 -> Sum/1
  Sum/1 -> contract/1
  rpw/1 -> expand rpw/1
  expand xyz/1 -> prod/2
  expand rpw/1 -> Sum/2
  crossprod/1 -> rotForceUnits/1
  contract/1 -> out/1

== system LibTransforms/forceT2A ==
  xyz : Inport  OutDataType=sfix(16)  OutScaling=2^0
  rpw : Inport  Port=2  OutDataType=sfix(16)  OutScaling=2^0
  DCM : Inport  Port=3  OutDataType=sfix(16)  OutScaling=2^0
  dir : Inport  Port=4  OutDataType=sfix(16)  OutScaling=2^0
  Mux1 : Mux  Inputs=2
  inverse force jacobian : LibTransforms/inverse force jacobian  SystemSampleTime=-1  dof=dof  rh=rh
  matrix inverse : LibTransforms/matrix inverse  SystemSampleTime=-1  rows=length(dof)  cols=size(rh, 2)  wate=fmax
  prod2 : Product  Multiplication=Matrix(*)  OutDataType=sfix(16)  OutScaling=2^0
  out : Outport  OutDataType=sfix(16)  OutScaling=2^0
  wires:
  matrix inverse/1 -> prod2/1
  dir/1 -> inverse force jacobian/1  "ebt_t"
  inverse force jacobian/1 -> matrix inverse/1
  DCM/1 -> inverse force jacobian/2
  prod2/1 -> out/1
  xyz/1 -> Mux1/1
  rpw/1 -> Mux1/2
  Mux1/1 -> prod2/2

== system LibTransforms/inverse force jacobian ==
  dir : Inport  OutDataType=sfix(16)  OutScaling=2^0
  DCM : Inport  Port=2  OutDataType=sfix(16)  OutScaling=2^0
  contract : Selector  NumberOfDimensions=2  InputPortWidth=3  IndexOptions=Index vector (dialog),Select all  Indices=dof,-1  OutputSizes=1
  matcat : Concatenate  Mode=Multidimensional array
  matrix cross product (column-wise) : LibTransforms/matrix cross product (column-wise)  SystemSampleTime=-1  cols=size(rh,2)
  prod1 : Product  Multiplication=Matrix(*)  OutDataType=sfix(16)  OutScaling=2^0
  rh : Constant  Value=rh  OutDataType=sfix(16)  OutScaling=2^0
  rotForceUnits : Gain  Gain=1/rotForceCanon  ParameterDataType=sfix(16)  ParameterScaling=2^0  OutDataType=sfix(16)  OutScaling=2^0
  t2w : Math  Operator=transpose  OutDataType=sfix(16)  OutScaling=2^0
  out : Outport  OutDataType=sfix(16)  OutScaling=2^0
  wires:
  contract/1 -> out/1
  matcat/1 -> contract/1
  rotForceUnits/1 -> matcat/2
  DCM/1 -> t2w/1
  dir/1 -> matrix cross product (column-wise)/2, prod1/2  "ebt_t"
  prod1/1 -> matcat/1  "ebt_w"
  rh/1 -> matrix cross product (column-wise)/1
  matrix cross product (column-wise)/1 -> rotForceUnits/1
  t2w/1 -> prod1/1

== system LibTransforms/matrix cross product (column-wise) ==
  A : Inport  OutDataType=sfix(16)  OutScaling=2^0
  B : Inport  Port=2  OutDataType=sfix(16)  OutScaling=2^0
  Assignment : Assignment  NumberOfDimensions=2  IndexOptions=Assign all,Index vector (port)  Indices=-1,1  OutputSizes=1,1
  For Iterator : ForIterator  IterationLimit=cols
  colA : Selector  NumberOfDimensions=2  InputPortWidth=3  IndexOptions=Select all,Index vector (port)  Indices=-1,-1  OutputSizes=1
  colB : Selector  NumberOfDimensions=2  InputPortWidth=3  IndexOptions=Select all,Index vector (port)  Indices=-1,-1  OutputSizes=1
  crossprod : aerospace/Axes Transformations/3x3 cross product  SystemSampleTime=-1
  zeros : Constant  Value=zeros(3,cols)  OutDataType=sfix(16)  OutScaling=2^0
  AxB : Outport  OutDataType=sfix(16)  OutScaling=2^0
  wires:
  colB/1 -> crossprod/2
  colA/1 -> crossprod/1
  crossprod/1 -> Assignment/2
  For Iterator/1 -> Assignment/3, colB/2, colA/2
  A/1 -> colA/1
  B/1 -> colB/1
  zeros/1 -> Assignment/1
  Assignment/1 -> AxB/1

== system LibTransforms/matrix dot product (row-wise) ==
  A : Inport  OutDataType=sfix(16)  OutScaling=2^0
  B : Inport  Port=2  OutDataType=sfix(16)  OutScaling=2^0
  Assignment : Assignment  IndexOptions=Index vector (port)  Indices=1  OutputSizes=[1 1]
  For Iterator : ForIterator  IterationLimit=rows
  dot product : simulink/Math Operations/Dot Product  InputSameDT=on  OutDataType=sfix(16)  OutScaling=2^-10  DoSatur=off
  rowA : Selector  NumberOfDimensions=2  InputPortWidth=3  IndexOptions=Index vector (port),Select all  Indices=-1,-1  OutputSizes=1
  rowB : Selector  NumberOfDimensions=2  InputPortWidth=3  IndexOptions=Index vector (port),Select all  Indices=-1,-1  OutputSizes=1
  zeros : Constant  Value=zeros(1,rows)  OutDataType=sfix(16)  OutScaling=2^0
  A*B : Outport  OutDataType=sfix(16)  OutScaling=2^0
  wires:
  dot product/1 -> Assignment/2
  rowB/1 -> dot product/2
  rowA/1 -> dot product/1
  B/1 -> rowB/1
  For Iterator/1 -> rowB/2, rowA/2, Assignment/3
  A/1 -> rowA/1
  zeros/1 -> Assignment/1
  Assignment/1 -> A*B/1

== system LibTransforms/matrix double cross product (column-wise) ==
  rotvel : Inport  OutDataType=sfix(16)  OutScaling=2^0
  ra : Inport  Port=2  OutDataType=sfix(16)  OutScaling=2^0
  ea : Inport  Port=3  OutDataType=sfix(16)  OutScaling=2^0
  Assignment : Assignment  IndexOptions=Index vector (port)  Indices=1  OutputSizes=[1 1]
  For Iterator : ForIterator  IterationLimit=cols
  col sel 1 : Selector  NumberOfDimensions=2  InputPortWidth=3  IndexOptions=Select all,Index vector (port)  Indices=-1,-1  OutputSizes=1
  col sel 2 : Selector  NumberOfDimensions=2  InputPortWidth=3  IndexOptions=Select all,Index vector (port)  Indices=-1,-1  OutputSizes=1
  crossprod1 : aerospace/Axes Transformations/3x3 cross product  SystemSampleTime=-1
  crossprod2 : aerospace/Axes Transformations/3x3 cross product  SystemSampleTime=-1
  dot product : simulink/Math Operations/Dot Product  InputSameDT=on  OutDataType=sfix(16)  OutScaling=2^-10  DoSatur=off
  zeros : Constant  Value=zeros(1,cols)  OutDataType=sfix(16)  OutScaling=2^0
  accel : Outport  OutDataType=sfix(16)  OutScaling=2^0
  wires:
  col sel 2/1 -> dot product/2
  ea/1 -> col sel 2/1
  dot product/1 -> Assignment/2
  crossprod2/1 -> dot product/1
  crossprod1/1 -> crossprod2/2
  col sel 1/1 -> crossprod1/2
  For Iterator/1 -> Assignment/3, col sel 1/2, col sel 2/2
  ra/1 -> col sel 1/1
  zeros/1 -> Assignment/1
  Assignment/1 -> accel/1
  rotvel/1 -> crossprod2/1, crossprod1/1

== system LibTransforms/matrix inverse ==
  inp : Inport  OutDataType=sfix(16)  OutScaling=2^0
  Multiport Switch : MultiPortSwitch  Inputs=3
  case : Constant  Value=c  OutDataType=sfix(16)  OutScaling=2^0
  rows < cols : Subsystem  TreatAsAtomicUnit=on
  rows == cols : Subsystem  TreatAsAtomicUnit=on
  rows > cols : Subsystem  TreatAsAtomicUnit=on
  switch case : SwitchCase  CaseConditions={1 2 3}  CaseShowDefault=off
  out : Outport  OutDataType=sfix(16)  OutScaling=2^0
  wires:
  Multiport Switch/1 -> out/1
  rows == cols/1(out) -> Multiport Switch/4
  rows > cols/1(out) -> Multiport Switch/3
  rows < cols/1(out) -> Multiport Switch/2
  inp/1 -> rows == cols/1(inp), rows < cols/1(inp), rows > cols/1(inp)
  case/1 -> Multiport Switch/1, switch case/1
  switch case/3 -> rows == cols/Action
  switch case/2 -> rows > cols/Action
  switch case/1 -> rows < cols/Action

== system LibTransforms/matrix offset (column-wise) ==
  inp : Inport  OutDataType=sfix(16)  OutScaling=2^0
  ofst : Inport  Port=2  OutDataType=sfix(16)  OutScaling=2^0
  Assignment : Assignment  NumberOfDimensions=2  IndexOptions=Assign all,Index vector (port)  Indices=-1,-1  OutputSizes=1,1
  For Iterator : ForIterator  IterationLimit=cols
  Sum : Sum  Inputs=|++  OutDataType=sfix(16)  OutScaling=2^0
  col sel : Selector  NumberOfDimensions=2  InputPortWidth=3  IndexOptions=Select all,Index vector (port)  Indices=-1,-1  OutputSizes=1
  zeros : Constant  Value=zeros(3,cols)  OutDataType=sfix(16)  OutScaling=2^0
  out : Outport  OutDataType=sfix(16)  OutScaling=2^0
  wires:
  col sel/1 -> Sum/1
  Sum/1 -> Assignment/2
  ofst/1 -> Sum/2
  For Iterator/1 -> col sel/2, Assignment/3
  inp/1 -> col sel/1
  zeros/1 -> Assignment/1
  Assignment/1 -> out/1

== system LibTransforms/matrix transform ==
  inp : Inport  OutDataType=sfix(16)  OutScaling=2^0
  constant : Constant  Value=matrix  OutDataType=sfix(16)  OutScaling=2^0
  product : Product  Multiplication=Matrix(*)  OutDataType=sfix(16)  OutScaling=2^0
  out : Outport  OutDataType=sfix(16)  OutScaling=2^0
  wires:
  inp/1 -> product/2
  product/1 -> out/1
  constant/1 -> product/1
